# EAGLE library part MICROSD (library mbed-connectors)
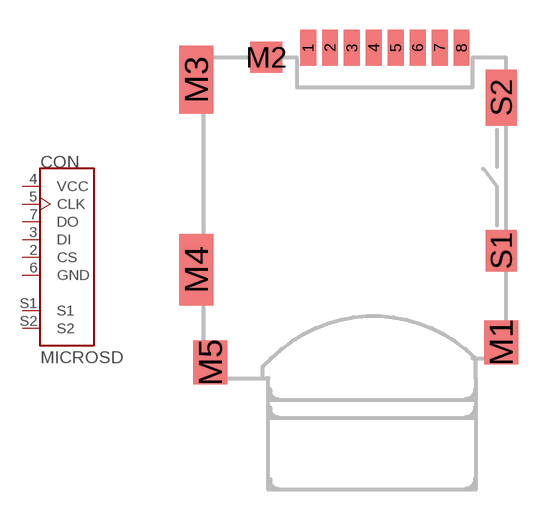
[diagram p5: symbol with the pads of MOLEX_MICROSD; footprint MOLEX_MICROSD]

Designator prefix CON

## MICROSDMOLEX_MIROSD  [MOLEX_MICROSD]
2  CS
3  DI
4  VCC  pas
5  CLK
6  GND  sup
7  DO
S1  S1
S2  S2

## Footprint MOLEX_MICROSD (pad centres in mm)
Molex 49225-0821 Micro-SD Connector
smd 0.8 x 1.8: 1 -3.89,10.66; 2 -2.79,10.66; 3 -1.69,10.66; 4 -0.59,10.66; 5 0.51,10.66; 6 1.61,10.66; 7 2.71,10.66; 8 3.81,10.66
smd 1.7 x 2.2: M1 5.8,-4.14; M5 -8.8,-5.14
smd 1.6 x 1.55: M2 -5.99,10.185
smd 1.7 x 3.4: M3 -9.5,9.06
smd 1.7 x 3.6: M4 -9.5,-0.49
smd 1.55 x 2.1: S1 5.8,0.46
smd 1.55 x 2.8: S2 5.8,8.16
